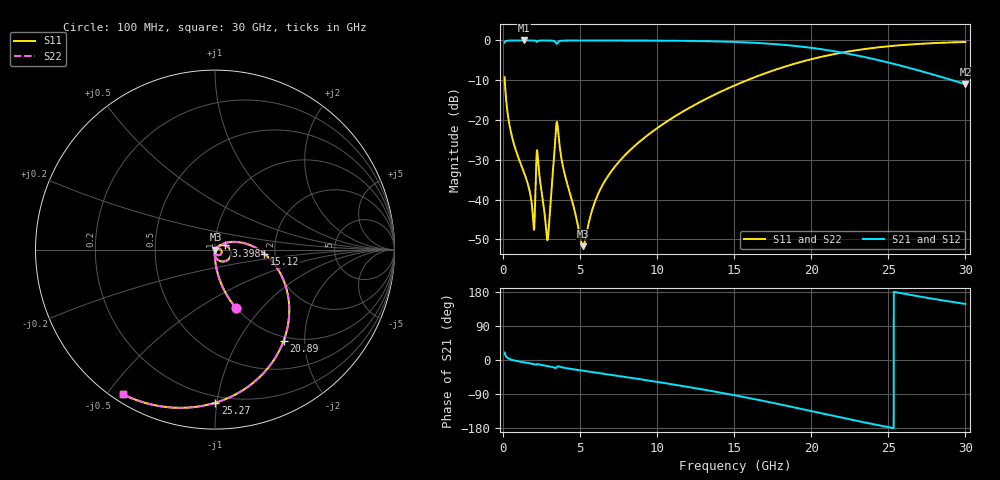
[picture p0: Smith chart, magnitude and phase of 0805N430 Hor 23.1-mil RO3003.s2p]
# GHz S MA R 50
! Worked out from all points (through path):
!   3201 points, 100 MHz to 30 GHz, reference 50 ohm
!   highest |S21| = -0.01 dB at 1.333 GHz (marker M1); lowest = -11.0 dB at 30 GHz (marker M2)
!   group delay of S21, straight-line fit = 20.6 ps
!   lowest |S11| = -51.7 dB at 5.183 GHz (marker M3), VSWR 1.01, Z = 50.2 - j0.116 ohm
!   |S11| at or under -10 dB: 109.9 MHz to 15.84 GHz (15.73 GHz wide, 197 % of centre)
!   |S22| runs from -51.7 to -0.4 dB; largest |S21 - S12| = 0
!   S11 on the Smith chart (normalised r, x): 100 MHz: 0.99, -0.73; 3.398 GHz: 1.12, +0.05; 15.12 GHz: 1.76, -0.09; 20.89 GHz: 0.93, -1.59; 25.27 GHz: 0.16, -0.99; 30 GHz: 0.03, -0.55
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0.1  0.3441 -70.4  0.9386 19.6  0.9386 19.6  0.3441 -70.4
0.5298125  0.06752 -88.5  0.9971 0.9  0.9971 0.9  0.06752 -88.5
1.333375  0.02255 -93.5  0.9987 -6.1  0.9987 -6.1  0.02255 -93.5
1.940719  0.006017 -75.9  0.9974 -10.4  0.9974 -10.4  0.006017 -75.9
2.286437  0.02812 -75.0  0.9872 -11.2  0.9872 -11.2  0.02812 -75.0
2.875094  0.00309 -26.6  0.9969 -15.8  0.9969 -15.8  0.00309 -26.6
3.005906  0.005861 32.0  0.996 -16.8  0.996 -16.8  0.005861 32.0
3.398344  0.06219 22.0  0.9536 -21.1  0.9536 -21.1  0.06219 22.0
3.566531  0.07499 -61.7  0.9455 -16.5  0.9455 -16.5  0.07499 -61.7
3.930938  0.0237 -95.1  0.9934 -20.3  0.9934 -20.3  0.0237 -95.1
5.089563  0.002809 -48.7  0.9972 -27.7  0.9972 -27.7  0.002809 -48.7
5.183  0.002599 -26.3  0.9972 -28.3  0.9972 -28.3  0.002599 -26.3
5.958531  0.009356 41.3  0.9972 -32.9  0.9972 -32.9  0.009356 41.3
6.762094  0.01915 44.4  0.997 -37.7  0.997 -37.7  0.01915 44.4
10.06978  0.08085 29.4  0.9931 -58.2  0.9931 -58.2  0.08085 29.4
15.05  0.2731 -4.3  0.9565 -93.3  0.9565 -93.3  0.2731 -4.3
15.11541  0.2766 -4.8  0.9555 -93.8  0.9555 -93.8  0.2766 -4.8
20.03956  0.5829 -45.7  0.8049 -135.1  0.8049 -135.1  0.5829 -45.7
20.88984  0.637 -53.2  0.763 -142.5  0.763 -142.5  0.637 -53.2
25.01978  0.8444 -87.9  0.5264 -177.4  0.5264 -177.4  0.8444 -87.9
25.27206  0.8534 -89.9  0.512 -179.4  0.512 -179.4  0.8534 -89.9
30  0.9562 -122.6  0.2815 147.9  0.2815 147.9  0.9562 -122.6
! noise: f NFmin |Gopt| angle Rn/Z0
0.1  0.0004467  0.865  0.7739  0.0007106
3.417  0.03383  0.9372  18.77  0.1169
6.743  0.01006  0.6518  36.46  0.004982
10.06  0.0137  0.6331  53.03  0.005694
13.39  0.01795  0.6379  68.5  0.00653
16.7  0.02306  0.6561  82.81  0.007432
20.03  0.02961  0.6849  96.27  0.00847
23.35  0.03843  0.7226  109.1  0.009716
26.67  0.05113  0.768  121.7  0.01123
30  0.07057  0.818  134.4  0.0129
